FUNCTION "Gest Avvisi/Allarmi" : VOID
TITLE =GESTIONE ALLARMI / AVVISI
AUTHOR : MassimoZ
VERSION : 0.1

BEGIN
NETWORK
TITLE ======== Avvisi Generali =======



NETWORK
TITLE =Avviso: Manca Marcia Generale
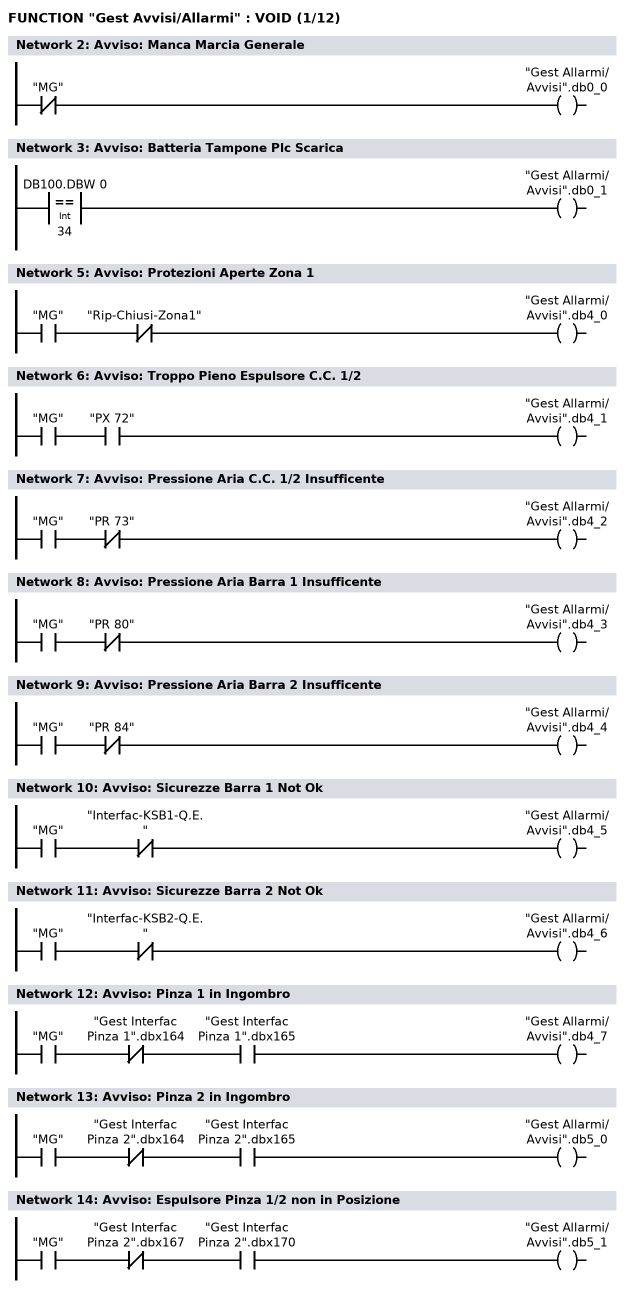
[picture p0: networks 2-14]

      UN    "MG";
      =     "Gest Allarmi/Avvisi".db0_0;
NETWORK
TITLE =Avviso: Batteria Tampone Plc Scarica

      L     DB100.DBW    0;
      L     34;
      ==I   ;
      =     "Gest Allarmi/Avvisi".db0_1;
NETWORK
TITLE ======== Avvisi Zona 1 =======



NETWORK
TITLE =Avviso: Protezioni Aperte Zona 1

      U     "MG";
      UN    "Rip-Chiusi-Zona1";
      =     "Gest Allarmi/Avvisi".db4_0;
NETWORK
TITLE =Avviso: Troppo Pieno Espulsore C.C. 1/2

      U     "MG";
      U     "PX 72";
      =     "Gest Allarmi/Avvisi".db4_1;
NETWORK
TITLE =Avviso: Pressione Aria C.C. 1/2 Insufficente

      U     "MG";
      UN    "PR 73";
      =     "Gest Allarmi/Avvisi".db4_2;
NETWORK
TITLE =Avviso: Pressione Aria Barra 1 Insufficente

      U     "MG";
      UN    "PR 80";
      =     "Gest Allarmi/Avvisi".db4_3;
NETWORK
TITLE =Avviso: Pressione Aria Barra 2 Insufficente

      U     "MG";
      UN    "PR 84";
      =     "Gest Allarmi/Avvisi".db4_4;
NETWORK
TITLE =Avviso: Sicurezze Barra 1 Not Ok

      U     "MG";
      UN    "Interfac-KSB1-Q.E.";
      =     "Gest Allarmi/Avvisi".db4_5;
NETWORK
TITLE =Avviso: Sicurezze Barra 2 Not Ok

      U     "MG";
      UN    "Interfac-KSB2-Q.E.";
      =     "Gest Allarmi/Avvisi".db4_6;
NETWORK
TITLE =Avviso: Pinza 1 in Ingombro

      U     "MG";
      UN    "Gest Interfac Pinza 1".dbx164;
      U     "Gest Interfac Pinza 1".dbx165;
      =     "Gest Allarmi/Avvisi".db4_7;
NETWORK
TITLE =Avviso: Pinza 2 in Ingombro

      U     "MG";
      UN    "Gest Interfac Pinza 2".dbx164;
      U     "Gest Interfac Pinza 2".dbx165;
      =     "Gest Allarmi/Avvisi".db5_0;
NETWORK
TITLE =Avviso: Espulsore Pinza 1/2 non in Posizione

      U     "MG";
      UN    "Gest Interfac Pinza 2".dbx167;
      U     "Gest Interfac Pinza 2".dbx170;
      =     "Gest Allarmi/Avvisi".db5_1;
NETWORK
TITLE =Avviso: Posa Coperchi in Ingombro
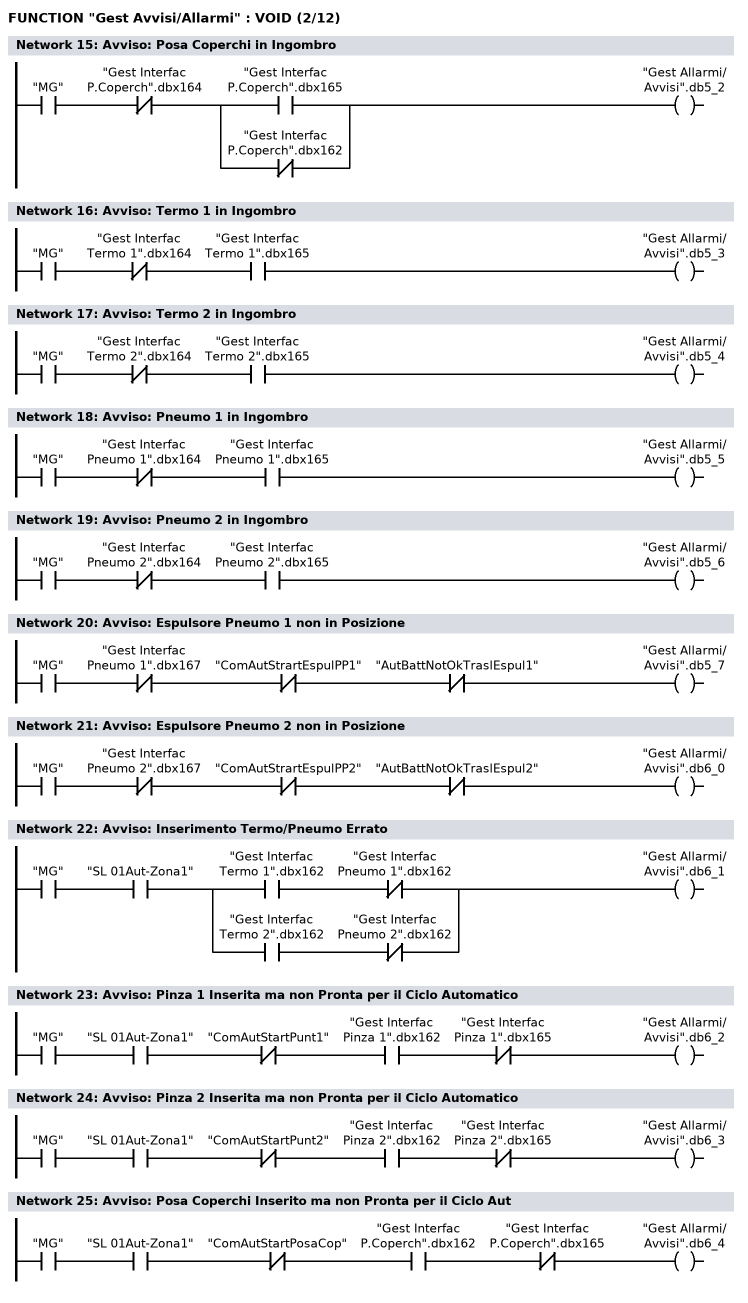
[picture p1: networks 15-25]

      U     "MG";
      UN    "Gest Interfac P.Coperch".dbx164;
      U(    ;
      O     "Gest Interfac P.Coperch".dbx165;
      ON    "Gest Interfac P.Coperch".dbx162;
      )     ;
      =     "Gest Allarmi/Avvisi".db5_2;
NETWORK
TITLE =Avviso: Termo 1 in Ingombro

      U     "MG";
      UN    "Gest Interfac Termo 1".dbx164;
      U     "Gest Interfac Termo 1".dbx165;
      =     "Gest Allarmi/Avvisi".db5_3;
NETWORK
TITLE =Avviso: Termo 2 in Ingombro

      U     "MG";
      UN    "Gest Interfac Termo 2".dbx164;
      U     "Gest Interfac Termo 2".dbx165;
      =     "Gest Allarmi/Avvisi".db5_4;
NETWORK
TITLE =Avviso: Pneumo 1 in Ingombro

      U     "MG";
      UN    "Gest Interfac Pneumo 1".dbx164;
      U     "Gest Interfac Pneumo 1".dbx165;
      =     "Gest Allarmi/Avvisi".db5_5;
NETWORK
TITLE =Avviso: Pneumo 2 in Ingombro

      U     "MG";
      UN    "Gest Interfac Pneumo 2".dbx164;
      U     "Gest Interfac Pneumo 2".dbx165;
      =     "Gest Allarmi/Avvisi".db5_6;
NETWORK
TITLE =Avviso: Espulsore Pneumo 1 non in Posizione

      U     "MG";
      UN    "Gest Interfac Pneumo 1".dbx167;
      UN    "ComAutStrartEspulPP1";
      UN    "AutBattNotOkTraslEspul1";
      =     "Gest Allarmi/Avvisi".db5_7;
NETWORK
TITLE =Avviso: Espulsore Pneumo 2 non in Posizione

      U     "MG";
      UN    "Gest Interfac Pneumo 2".dbx167;
      UN    "ComAutStrartEspulPP2";
      UN    "AutBattNotOkTraslEspul2";
      =     "Gest Allarmi/Avvisi".db6_0;
NETWORK
TITLE =Avviso: Inserimento Termo/Pneumo Errato

      U     "MG";
      U     "SL 01Aut-Zona1";
      U(    ;
      U     "Gest Interfac Termo 1".dbx162;
      UN    "Gest Interfac Pneumo 1".dbx162;
      O     ;
      U     "Gest Interfac Termo 2".dbx162;
      UN    "Gest Interfac Pneumo 2".dbx162;
      )     ;
      =     "Gest Allarmi/Avvisi".db6_1;
NETWORK
TITLE =Avviso: Pinza 1 Inserita ma non Pronta per il Ciclo Automatico

      U     "MG";
      U     "SL 01Aut-Zona1";
      UN    "ComAutStartPunt1";
      U     "Gest Interfac Pinza 1".dbx162;
      UN    "Gest Interfac Pinza 1".dbx165;
      =     "Gest Allarmi/Avvisi".db6_2;
NETWORK
TITLE =Avviso: Pinza 2 Inserita ma non Pronta per il Ciclo Automatico

      U     "MG";
      U     "SL 01Aut-Zona1";
      UN    "ComAutStartPunt2";
      U     "Gest Interfac Pinza 2".dbx162;
      UN    "Gest Interfac Pinza 2".dbx165;
      =     "Gest Allarmi/Avvisi".db6_3;
NETWORK
TITLE =Avviso: Posa Coperchi Inserito ma non Pronta per il Ciclo Aut

      U     "MG";
      U     "SL 01Aut-Zona1";
      UN    "ComAutStartPosaCop";
      U     "Gest Interfac P.Coperch".dbx162;
      UN    "Gest Interfac P.Coperch".dbx165;
      =     "Gest Allarmi/Avvisi".db6_4;
NETWORK
TITLE =Avviso: Termo 1 Inserita ma non Pronta per il Ciclo Automatico
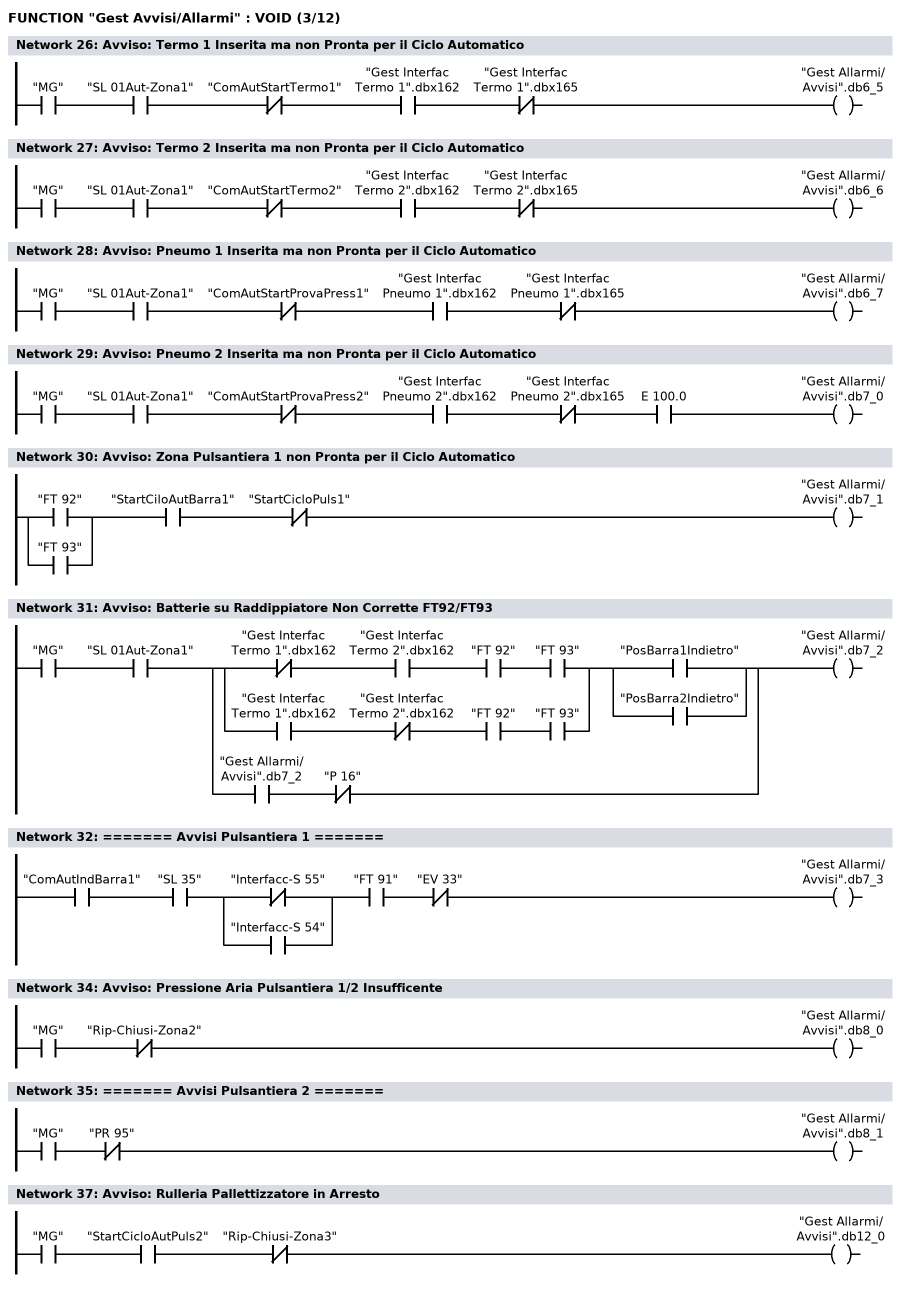
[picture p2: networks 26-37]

      U     "MG";
      U     "SL 01Aut-Zona1";
      UN    "ComAutStartTermo1";
      U     "Gest Interfac Termo 1".dbx162;
      UN    "Gest Interfac Termo 1".dbx165;
      =     "Gest Allarmi/Avvisi".db6_5;
NETWORK
TITLE =Avviso: Termo 2 Inserita ma non Pronta per il Ciclo Automatico

      U     "MG";
      U     "SL 01Aut-Zona1";
      UN    "ComAutStartTermo2";
      U     "Gest Interfac Termo 2".dbx162;
      UN    "Gest Interfac Termo 2".dbx165;
      =     "Gest Allarmi/Avvisi".db6_6;
NETWORK
TITLE =Avviso: Pneumo 1 Inserita ma non Pronta per il Ciclo Automatico

      U     "MG";
      U     "SL 01Aut-Zona1";
      UN    "ComAutStartProvaPress1";
      U     "Gest Interfac Pneumo 1".dbx162;
      UN    "Gest Interfac Pneumo 1".dbx165;
      =     "Gest Allarmi/Avvisi".db6_7;
NETWORK
TITLE =Avviso: Pneumo 2 Inserita ma non Pronta per il Ciclo Automatico

      U     "MG";
      U     "SL 01Aut-Zona1";
      UN    "ComAutStartProvaPress2";
      U     "Gest Interfac Pneumo 2".dbx162;
      UN    "Gest Interfac Pneumo 2".dbx165;
      U     E    100.0;
      =     "Gest Allarmi/Avvisi".db7_0;
NETWORK
TITLE =Avviso: Zona Pulsantiera 1 non Pronta per il Ciclo Automatico

      U(    ;
      O     "FT 92";
      O     "FT 93";
      )     ;
      U     "StartCiloAutBarra1";
      UN    "StartCicloPuls1";
      =     "Gest Allarmi/Avvisi".db7_1;
NETWORK
TITLE =Avviso: Batterie su Raddippiatore Non Corrette FT92/FT93

      U     "MG";
      U     "SL 01Aut-Zona1";
      U(    ;
      U(    ;
      UN    "Gest Interfac Termo 1".dbx162;
      U     "Gest Interfac Termo 2".dbx162;
      U     "FT 92";
      U     "FT 93";
      O     ;
      U     "Gest Interfac Termo 1".dbx162;
      UN    "Gest Interfac Termo 2".dbx162;
      U     "FT 92";
      U     "FT 93";
      )     ;
      U(    ;
      O     "PosBarra1Indietro";
      O     "PosBarra2Indietro";
      )     ;
      O     ;
      U     "Gest Allarmi/Avvisi".db7_2;
      UN    "P 16";
      )     ;
      =     "Gest Allarmi/Avvisi".db7_2;
NETWORK
TITLE ======== Avvisi Pulsantiera 1 =======



      U     "ComAutIndBarra1";
      U     "SL 35";
      U(    ;
      ON    "Interfacc-S 55";
      O     "Interfacc-S 54";
      )     ;
      U     "FT 91";
      UN    "EV 33";
      =     "Gest Allarmi/Avvisi".db7_3;
NETWORK
TITLE =Avviso: Protezioni Aperte Pulsantiera 1

NETWORK
TITLE =Avviso: Pressione Aria Pulsantiera 1/2 Insufficente

      U     "MG";
      UN    "Rip-Chiusi-Zona2";
      =     "Gest Allarmi/Avvisi".db8_0;
NETWORK
TITLE ======== Avvisi Pulsantiera 2 =======



      U     "MG";
      UN    "PR 95";
      =     "Gest Allarmi/Avvisi".db8_1;
NETWORK
TITLE =Avviso: Protezioni Aperte Pulsantiera 2

NETWORK
TITLE =Avviso: Rulleria Pallettizzatore in Arresto

      U     "MG";
      U     "StartCicloAutPuls2";
      UN    "Rip-Chiusi-Zona3";
      =     "Gest Allarmi/Avvisi".db12_0;
NETWORK
TITLE =Avviso: Troppo Pieno Rulleria Pallettizzatore
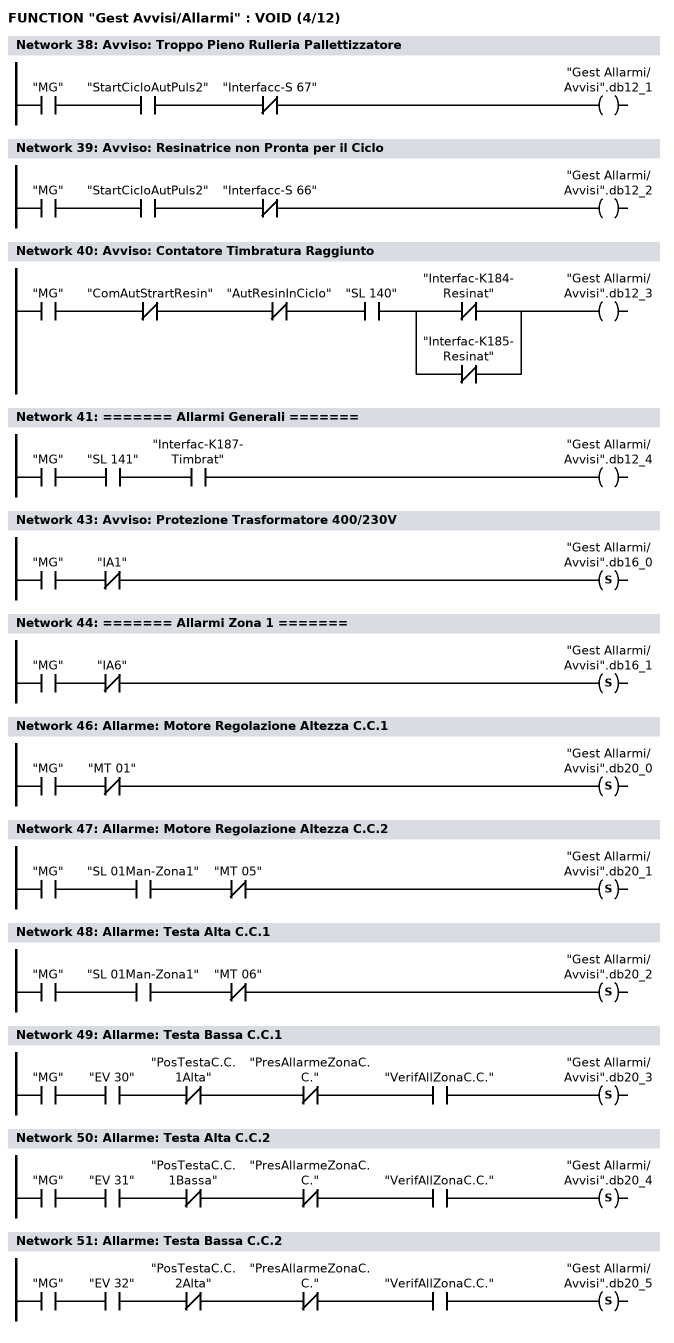
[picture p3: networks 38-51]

      U     "MG";
      U     "StartCicloAutPuls2";
      UN    "Interfacc-S 67";
      =     "Gest Allarmi/Avvisi".db12_1;
NETWORK
TITLE =Avviso: Resinatrice non Pronta per il Ciclo

      U     "MG";
      U     "StartCicloAutPuls2";
      UN    "Interfacc-S 66";
      =     "Gest Allarmi/Avvisi".db12_2;
NETWORK
TITLE =Avviso: Contatore Timbratura Raggiunto

      U     "MG";
      UN    "ComAutStrartResin";
      UN    "AutResinInCiclo";
      U     "SL 140";
      U(    ;
      ON    "Interfac-K184-Resinat";
      ON    "Interfac-K185-Resinat";
      )     ;
      =     "Gest Allarmi/Avvisi".db12_3;
NETWORK
TITLE ======== Allarmi Generali =======



      U     "MG";
      U     "SL 141";
      U     "Interfac-K187-Timbrat";
      =     "Gest Allarmi/Avvisi".db12_4;
NETWORK
TITLE =Avviso: Alimentazione Quadro Elettrico

NETWORK
TITLE =Avviso: Protezione Trasformatore 400/230V

      U     "MG";
      UN    "IA1";
      S     "Gest Allarmi/Avvisi".db16_0;
NETWORK
TITLE ======== Allarmi Zona 1 =======



      U     "MG";
      UN    "IA6";
      S     "Gest Allarmi/Avvisi".db16_1;
NETWORK
TITLE =Allarme: Motore Nastro 1

NETWORK
TITLE =Allarme: Motore Regolazione Altezza C.C.1

      U     "MG";
      UN    "MT 01";
      S     "Gest Allarmi/Avvisi".db20_0;
NETWORK
TITLE =Allarme: Motore Regolazione Altezza C.C.2

      U     "MG";
      U     "SL 01Man-Zona1";
      UN    "MT 05";
      S     "Gest Allarmi/Avvisi".db20_1;
NETWORK
TITLE =Allarme: Testa Alta C.C.1

      U     "MG";
      U     "SL 01Man-Zona1";
      UN    "MT 06";
      S     "Gest Allarmi/Avvisi".db20_2;
NETWORK
TITLE =Allarme: Testa Bassa C.C.1

      U     "MG";
      U     "EV 30";
      UN    "PosTestaC.C.1Alta";
      UN    "PresAllarmeZonaC.C.";
      U     "VerifAllZonaC.C.";
      S     "Gest Allarmi/Avvisi".db20_3;
NETWORK
TITLE =Allarme: Testa Alta C.C.2

      U     "MG";
      U     "EV 31";
      UN    "PosTestaC.C.1Bassa";
      UN    "PresAllarmeZonaC.C.";
      U     "VerifAllZonaC.C.";
      S     "Gest Allarmi/Avvisi".db20_4;
NETWORK
TITLE =Allarme: Testa Bassa C.C.2

      U     "MG";
      U     "EV 32";
      UN    "PosTestaC.C.2Alta";
      UN    "PresAllarmeZonaC.C.";
      U     "VerifAllZonaC.C.";
      S     "Gest Allarmi/Avvisi".db20_5;
NETWORK
TITLE =Allarme: Parzializzatore Inizio Linea Aperto
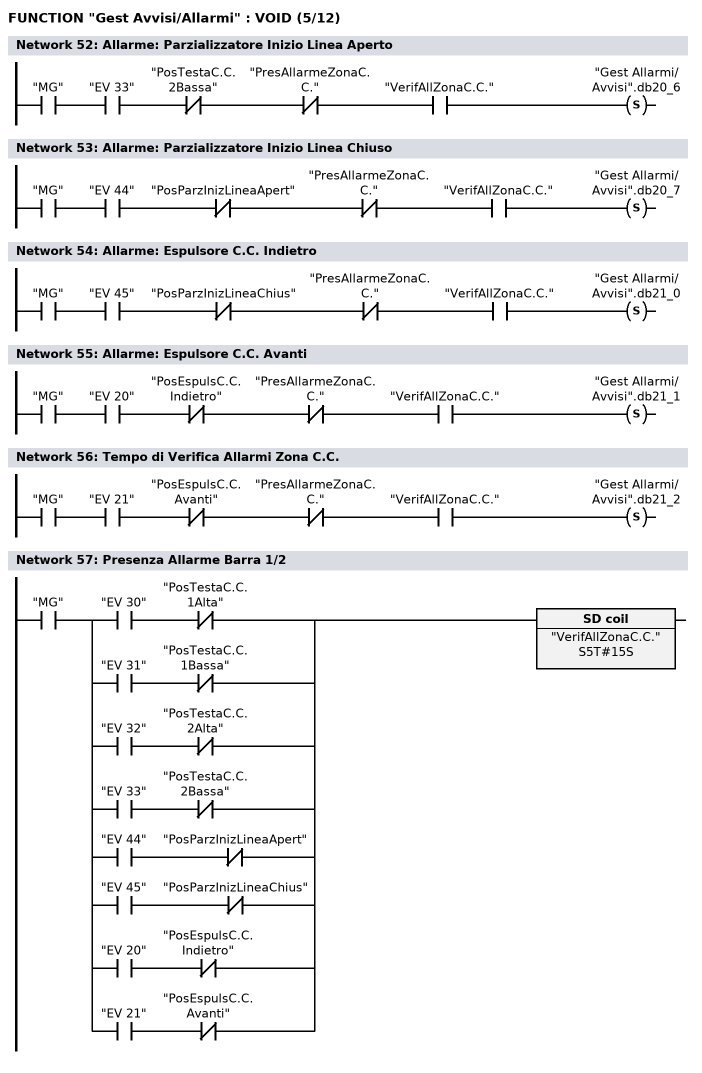
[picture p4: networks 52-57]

      U     "MG";
      U     "EV 33";
      UN    "PosTestaC.C.2Bassa";
      UN    "PresAllarmeZonaC.C.";
      U     "VerifAllZonaC.C.";
      S     "Gest Allarmi/Avvisi".db20_6;
NETWORK
TITLE =Allarme: Parzializzatore Inizio Linea Chiuso

      U     "MG";
      U     "EV 44";
      UN    "PosParzInizLineaApert";
      UN    "PresAllarmeZonaC.C.";
      U     "VerifAllZonaC.C.";
      S     "Gest Allarmi/Avvisi".db20_7;
NETWORK
TITLE =Allarme: Espulsore C.C. Indietro

      U     "MG";
      U     "EV 45";
      UN    "PosParzInizLineaChius";
      UN    "PresAllarmeZonaC.C.";
      U     "VerifAllZonaC.C.";
      S     "Gest Allarmi/Avvisi".db21_0;
NETWORK
TITLE =Allarme: Espulsore C.C. Avanti

      U     "MG";
      U     "EV 20";
      UN    "PosEspulsC.C.Indietro";
      UN    "PresAllarmeZonaC.C.";
      U     "VerifAllZonaC.C.";
      S     "Gest Allarmi/Avvisi".db21_1;
NETWORK
TITLE =Tempo di Verifica Allarmi Zona C.C.

      U     "MG";
      U     "EV 21";
      UN    "PosEspulsC.C.Avanti";
      UN    "PresAllarmeZonaC.C.";
      U     "VerifAllZonaC.C.";
      S     "Gest Allarmi/Avvisi".db21_2;
NETWORK
TITLE =Presenza Allarme Barra 1/2

      U     "MG";
      U(    ;
      U     "EV 30";
      UN    "PosTestaC.C.1Alta";
      O     ;
      U     "EV 31";
      UN    "PosTestaC.C.1Bassa";
      O     ;
      U     "EV 32";
      UN    "PosTestaC.C.2Alta";
      O     ;
      U     "EV 33";
      UN    "PosTestaC.C.2Bassa";
      O     ;
      U     "EV 44";
      UN    "PosParzInizLineaApert";
      O     ;
      U     "EV 45";
      UN    "PosParzInizLineaChius";
      O     ;
      U     "EV 20";
      UN    "PosEspulsC.C.Indietro";
      O     ;
      U     "EV 21";
      UN    "PosEspulsC.C.Avanti";
      )     ;
      L     S5T#15S;
      SE    "VerifAllZonaC.C.";
NETWORK
TITLE =Allarme: Barra 1 Indietro
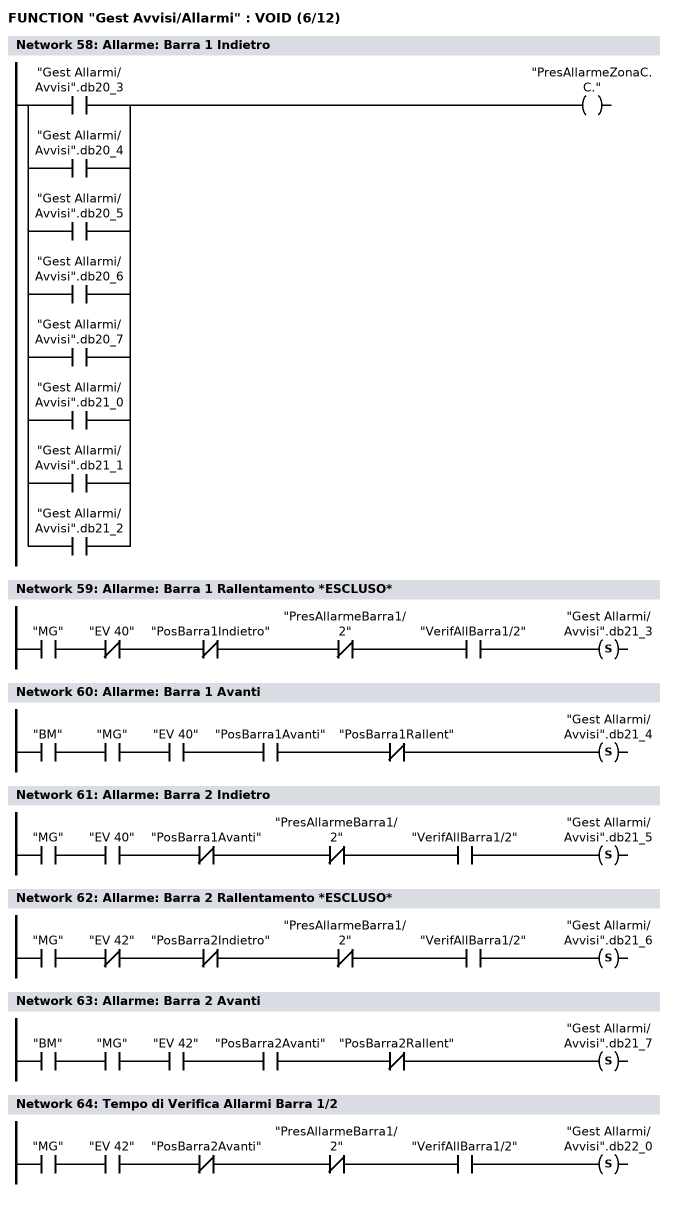
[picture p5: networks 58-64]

      O     "Gest Allarmi/Avvisi".db20_3;
      O     "Gest Allarmi/Avvisi".db20_4;
      O     "Gest Allarmi/Avvisi".db20_5;
      O     "Gest Allarmi/Avvisi".db20_6;
      O     "Gest Allarmi/Avvisi".db20_7;
      O     "Gest Allarmi/Avvisi".db21_0;
      O     "Gest Allarmi/Avvisi".db21_1;
      O     "Gest Allarmi/Avvisi".db21_2;
      =     "PresAllarmeZonaC.C.";
NETWORK
TITLE =Allarme: Barra 1 Rallentamento *ESCLUSO*

      U     "MG";
      UN    "EV 40";
      UN    "PosBarra1Indietro";
      UN    "PresAllarmeBarra1/2";
      U     "VerifAllBarra1/2";
      S     "Gest Allarmi/Avvisi".db21_3;
NETWORK
TITLE =Allarme: Barra 1 Avanti

      U     "BM";
      U     "MG";
      U     "EV 40";
      U     "PosBarra1Avanti";
      UN    "PosBarra1Rallent";
      S     "Gest Allarmi/Avvisi".db21_4;
NETWORK
TITLE =Allarme: Barra 2 Indietro

      U     "MG";
      U     "EV 40";
      UN    "PosBarra1Avanti";
      UN    "PresAllarmeBarra1/2";
      U     "VerifAllBarra1/2";
      S     "Gest Allarmi/Avvisi".db21_5;
NETWORK
TITLE =Allarme: Barra 2 Rallentamento *ESCLUSO*

      U     "MG";
      UN    "EV 42";
      UN    "PosBarra2Indietro";
      UN    "PresAllarmeBarra1/2";
      U     "VerifAllBarra1/2";
      S     "Gest Allarmi/Avvisi".db21_6;
NETWORK
TITLE =Allarme: Barra 2 Avanti

      U     "BM";
      U     "MG";
      U     "EV 42";
      U     "PosBarra2Avanti";
      UN    "PosBarra2Rallent";
      S     "Gest Allarmi/Avvisi".db21_7;
NETWORK
TITLE =Tempo di Verifica Allarmi Barra 1/2

      U     "MG";
      U     "EV 42";
      UN    "PosBarra2Avanti";
      UN    "PresAllarmeBarra1/2";
      U     "VerifAllBarra1/2";
      S     "Gest Allarmi/Avvisi".db22_0;
NETWORK
TITLE =Presenza Allarme Barra 1/2
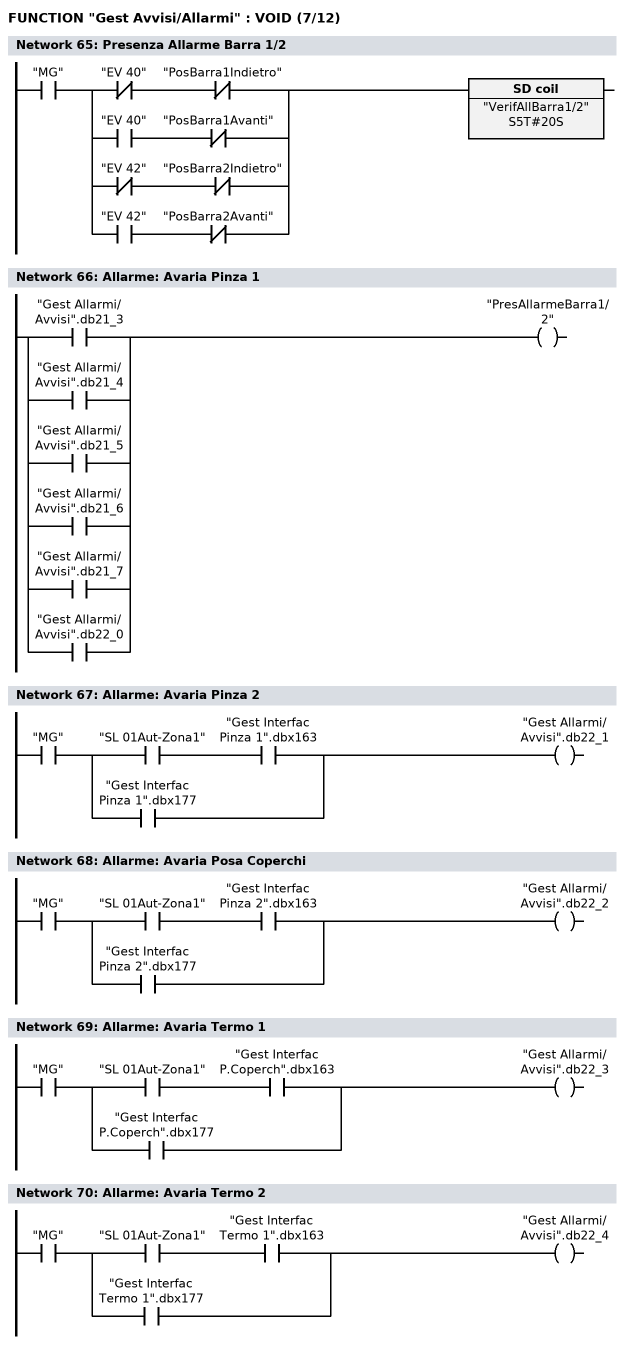
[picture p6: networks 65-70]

      U     "MG";
      U(    ;
      UN    "EV 40";
      UN    "PosBarra1Indietro";
      O     ;
      U     "EV 40";
      UN    "PosBarra1Avanti";
      O     ;
      UN    "EV 42";
      UN    "PosBarra2Indietro";
      O     ;
      U     "EV 42";
      UN    "PosBarra2Avanti";
      )     ;
      L     S5T#20S;
      SE    "VerifAllBarra1/2";
NETWORK
TITLE =Allarme: Avaria Pinza 1

      O     "Gest Allarmi/Avvisi".db21_3;
      O     "Gest Allarmi/Avvisi".db21_4;
      O     "Gest Allarmi/Avvisi".db21_5;
      O     "Gest Allarmi/Avvisi".db21_6;
      O     "Gest Allarmi/Avvisi".db21_7;
      O     "Gest Allarmi/Avvisi".db22_0;
      =     "PresAllarmeBarra1/2";
NETWORK
TITLE =Allarme: Avaria Pinza 2

      U     "MG";
      U(    ;
      U     "SL 01Aut-Zona1";
      U     "Gest Interfac Pinza 1".dbx163;
      O     "Gest Interfac Pinza 1".dbx177;
      )     ;
      =     "Gest Allarmi/Avvisi".db22_1;
NETWORK
TITLE =Allarme: Avaria Posa Coperchi

      U     "MG";
      U(    ;
      U     "SL 01Aut-Zona1";
      U     "Gest Interfac Pinza 2".dbx163;
      O     "Gest Interfac Pinza 2".dbx177;
      )     ;
      =     "Gest Allarmi/Avvisi".db22_2;
NETWORK
TITLE =Allarme: Avaria Termo 1

      U     "MG";
      U(    ;
      U     "SL 01Aut-Zona1";
      U     "Gest Interfac P.Coperch".dbx163;
      O     "Gest Interfac P.Coperch".dbx177;
      )     ;
      =     "Gest Allarmi/Avvisi".db22_3;
NETWORK
TITLE =Allarme: Avaria Termo 2

      U     "MG";
      U(    ;
      U     "SL 01Aut-Zona1";
      U     "Gest Interfac Termo 1".dbx163;
      O     "Gest Interfac Termo 1".dbx177;
      )     ;
      =     "Gest Allarmi/Avvisi".db22_4;
NETWORK
TITLE =Allarme: Avaria Pneumo 1
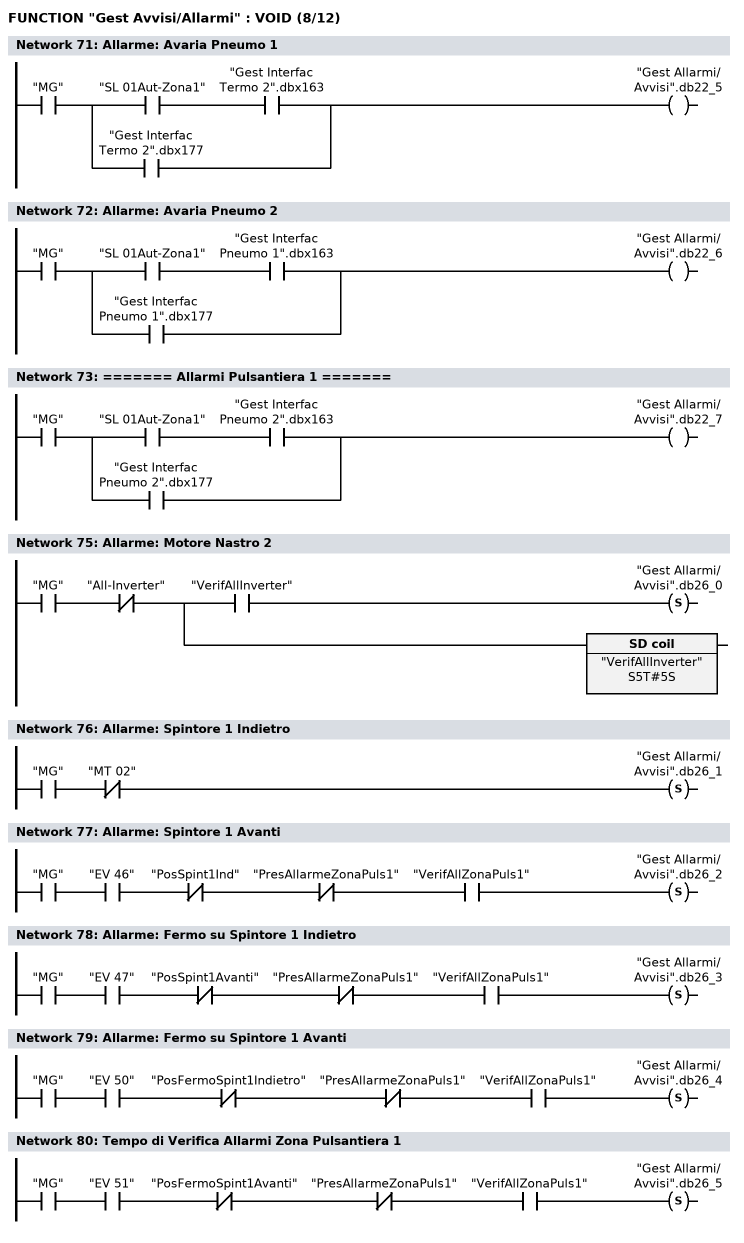
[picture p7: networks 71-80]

      U     "MG";
      U(    ;
      U     "SL 01Aut-Zona1";
      U     "Gest Interfac Termo 2".dbx163;
      O     "Gest Interfac Termo 2".dbx177;
      )     ;
      =     "Gest Allarmi/Avvisi".db22_5;
NETWORK
TITLE =Allarme: Avaria Pneumo 2

      U     "MG";
      U(    ;
      U     "SL 01Aut-Zona1";
      U     "Gest Interfac Pneumo 1".dbx163;
      O     "Gest Interfac Pneumo 1".dbx177;
      )     ;
      =     "Gest Allarmi/Avvisi".db22_6;
NETWORK
TITLE ======== Allarmi Pulsantiera 1 =======



      U     "MG";
      U(    ;
      U     "SL 01Aut-Zona1";
      U     "Gest Interfac Pneumo 2".dbx163;
      O     "Gest Interfac Pneumo 2".dbx177;
      )     ;
      =     "Gest Allarmi/Avvisi".db22_7;
NETWORK
TITLE =Allarme: Inverter

NETWORK
TITLE =Allarme: Motore Nastro 2

      U     "MG";
      UN    "All-Inverter";
      =     L      0.0;
      U     L      0.0;
      U     "VerifAllInverter";
      S     "Gest Allarmi/Avvisi".db26_0;
      U     L      0.0;
      BLD   102;
      L     S5T#5S;
      SE    "VerifAllInverter";
NETWORK
TITLE =Allarme: Spintore 1 Indietro

      U     "MG";
      UN    "MT 02";
      S     "Gest Allarmi/Avvisi".db26_1;
NETWORK
TITLE =Allarme: Spintore 1 Avanti

      U     "MG";
      U     "EV 46";
      UN    "PosSpint1Ind";
      UN    "PresAllarmeZonaPuls1";
      U     "VerifAllZonaPuls1";
      S     "Gest Allarmi/Avvisi".db26_2;
NETWORK
TITLE =Allarme: Fermo su Spintore 1 Indietro

      U     "MG";
      U     "EV 47";
      UN    "PosSpint1Avanti";
      UN    "PresAllarmeZonaPuls1";
      U     "VerifAllZonaPuls1";
      S     "Gest Allarmi/Avvisi".db26_3;
NETWORK
TITLE =Allarme: Fermo su Spintore 1 Avanti

      U     "MG";
      U     "EV 50";
      UN    "PosFermoSpint1Indietro";
      UN    "PresAllarmeZonaPuls1";
      U     "VerifAllZonaPuls1";
      S     "Gest Allarmi/Avvisi".db26_4;
NETWORK
TITLE =Tempo di Verifica Allarmi Zona Pulsantiera 1

      U     "MG";
      U     "EV 51";
      UN    "PosFermoSpint1Avanti";
      UN    "PresAllarmeZonaPuls1";
      U     "VerifAllZonaPuls1";
      S     "Gest Allarmi/Avvisi".db26_5;
NETWORK
TITLE =Presenza Allarme Zona Pulsantiera 1
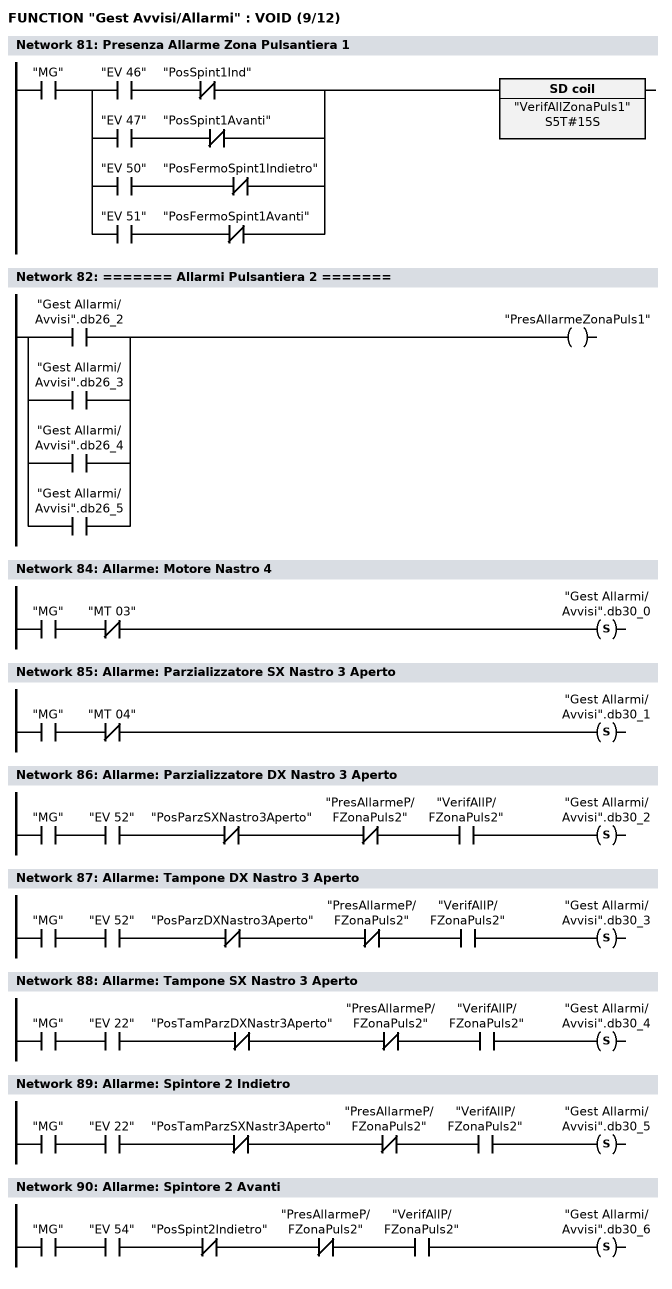
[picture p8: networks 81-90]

      U     "MG";
      U(    ;
      U     "EV 46";
      UN    "PosSpint1Ind";
      O     ;
      U     "EV 47";
      UN    "PosSpint1Avanti";
      O     ;
      U     "EV 50";
      UN    "PosFermoSpint1Indietro";
      O     ;
      U     "EV 51";
      UN    "PosFermoSpint1Avanti";
      )     ;
      L     S5T#15S;
      SE    "VerifAllZonaPuls1";
NETWORK
TITLE ======== Allarmi Pulsantiera 2 =======



      O     "Gest Allarmi/Avvisi".db26_2;
      O     "Gest Allarmi/Avvisi".db26_3;
      O     "Gest Allarmi/Avvisi".db26_4;
      O     "Gest Allarmi/Avvisi".db26_5;
      =     "PresAllarmeZonaPuls1";
NETWORK
TITLE =Allarme: Motore Nastro 3

NETWORK
TITLE =Allarme: Motore Nastro 4

      U     "MG";
      UN    "MT 03";
      S     "Gest Allarmi/Avvisi".db30_0;
NETWORK
TITLE =Allarme: Parzializzatore SX Nastro 3 Aperto

      U     "MG";
      UN    "MT 04";
      S     "Gest Allarmi/Avvisi".db30_1;
NETWORK
TITLE =Allarme: Parzializzatore DX Nastro 3 Aperto

      U     "MG";
      U     "EV 52";
      UN    "PosParzSXNastro3Aperto";
      UN    "PresAllarmeP/FZonaPuls2";
      U     "VerifAllP/FZonaPuls2";
      S     "Gest Allarmi/Avvisi".db30_2;
NETWORK
TITLE =Allarme: Tampone DX Nastro 3 Aperto

      U     "MG";
      U     "EV 52";
      UN    "PosParzDXNastro3Aperto";
      UN    "PresAllarmeP/FZonaPuls2";
      U     "VerifAllP/FZonaPuls2";
      S     "Gest Allarmi/Avvisi".db30_3;
NETWORK
TITLE =Allarme: Tampone SX Nastro 3 Aperto

      U     "MG";
      U     "EV 22";
      UN    "PosTamParzDXNastr3Aperto";
      UN    "PresAllarmeP/FZonaPuls2";
      U     "VerifAllP/FZonaPuls2";
      S     "Gest Allarmi/Avvisi".db30_4;
NETWORK
TITLE =Allarme: Spintore 2 Indietro

      U     "MG";
      U     "EV 22";
      UN    "PosTamParzSXNastr3Aperto";
      UN    "PresAllarmeP/FZonaPuls2";
      U     "VerifAllP/FZonaPuls2";
      S     "Gest Allarmi/Avvisi".db30_5;
NETWORK
TITLE =Allarme: Spintore 2 Avanti

      U     "MG";
      U     "EV 54";
      UN    "PosSpint2Indietro";
      UN    "PresAllarmeP/FZonaPuls2";
      U     "VerifAllP/FZonaPuls2";
      S     "Gest Allarmi/Avvisi".db30_6;
NETWORK
TITLE =Allarme: Fermo Anteriore Resinatrice Aperto
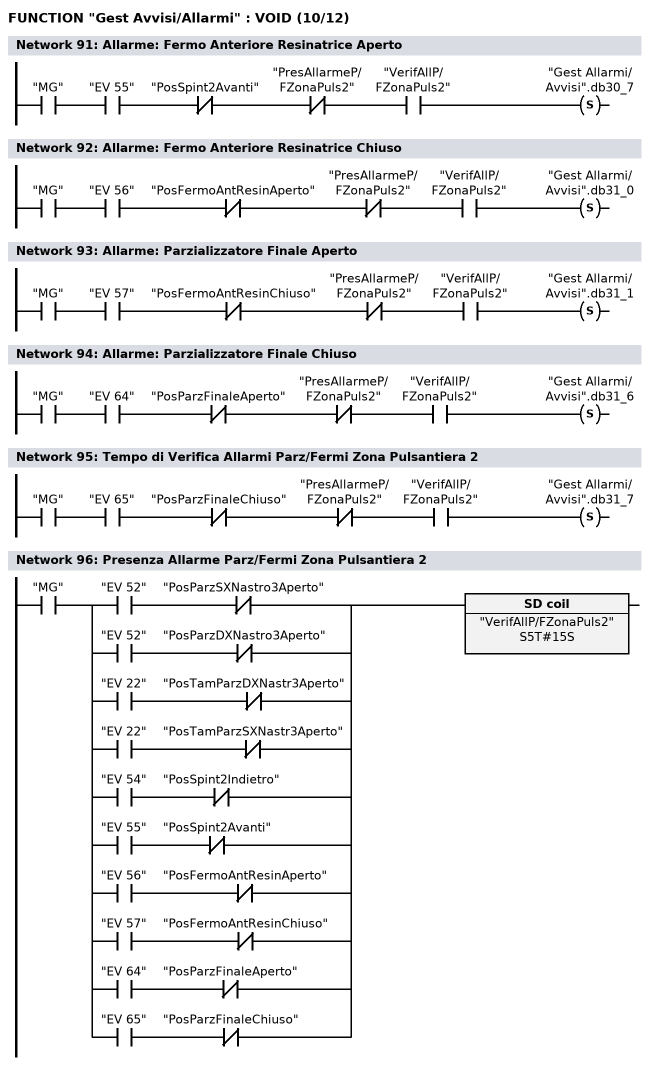
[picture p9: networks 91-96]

      U     "MG";
      U     "EV 55";
      UN    "PosSpint2Avanti";
      UN    "PresAllarmeP/FZonaPuls2";
      U     "VerifAllP/FZonaPuls2";
      S     "Gest Allarmi/Avvisi".db30_7;
NETWORK
TITLE =Allarme: Fermo Anteriore Resinatrice Chiuso

      U     "MG";
      U     "EV 56";
      UN    "PosFermoAntResinAperto";
      UN    "PresAllarmeP/FZonaPuls2";
      U     "VerifAllP/FZonaPuls2";
      S     "Gest Allarmi/Avvisi".db31_0;
NETWORK
TITLE =Allarme: Parzializzatore Finale Aperto

      U     "MG";
      U     "EV 57";
      UN    "PosFermoAntResinChiuso";
      UN    "PresAllarmeP/FZonaPuls2";
      U     "VerifAllP/FZonaPuls2";
      S     "Gest Allarmi/Avvisi".db31_1;
NETWORK
TITLE =Allarme: Parzializzatore Finale Chiuso

      U     "MG";
      U     "EV 64";
      UN    "PosParzFinaleAperto";
      UN    "PresAllarmeP/FZonaPuls2";
      U     "VerifAllP/FZonaPuls2";
      S     "Gest Allarmi/Avvisi".db31_6;
NETWORK
TITLE =Tempo di Verifica Allarmi Parz/Fermi Zona Pulsantiera 2

      U     "MG";
      U     "EV 65";
      UN    "PosParzFinaleChiuso";
      UN    "PresAllarmeP/FZonaPuls2";
      U     "VerifAllP/FZonaPuls2";
      S     "Gest Allarmi/Avvisi".db31_7;
NETWORK
TITLE =Presenza Allarme Parz/Fermi Zona Pulsantiera 2

      U     "MG";
      U(    ;
      U     "EV 52";
      UN    "PosParzSXNastro3Aperto";
      O     ;
      U     "EV 52";
      UN    "PosParzDXNastro3Aperto";
      O     ;
      U     "EV 22";
      UN    "PosTamParzDXNastr3Aperto";
      O     ;
      U     "EV 22";
      UN    "PosTamParzSXNastr3Aperto";
      O     ;
      U     "EV 54";
      UN    "PosSpint2Indietro";
      O     ;
      U     "EV 55";
      UN    "PosSpint2Avanti";
      O     ;
      U     "EV 56";
      UN    "PosFermoAntResinAperto";
      O     ;
      U     "EV 57";
      UN    "PosFermoAntResinChiuso";
      O     ;
      U     "EV 64";
      UN    "PosParzFinaleAperto";
      O     ;
      U     "EV 65";
      UN    "PosParzFinaleChiuso";
      )     ;
      L     S5T#15S;
      SE    "VerifAllP/FZonaPuls2";
NETWORK
TITLE =Allarme: Fermo Resinatrice Aperto
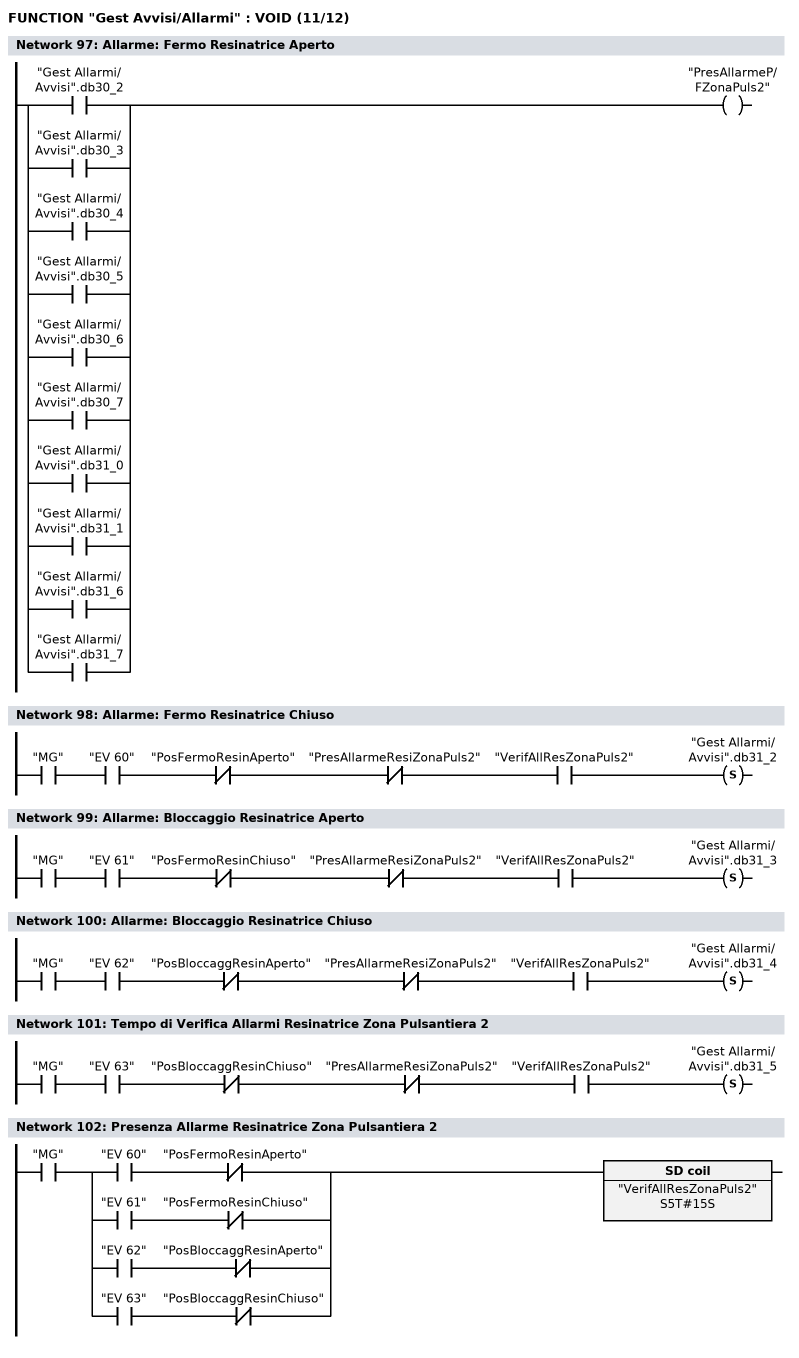
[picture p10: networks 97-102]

      O     "Gest Allarmi/Avvisi".db30_2;
      O     "Gest Allarmi/Avvisi".db30_3;
      O     "Gest Allarmi/Avvisi".db30_4;
      O     "Gest Allarmi/Avvisi".db30_5;
      O     "Gest Allarmi/Avvisi".db30_6;
      O     "Gest Allarmi/Avvisi".db30_7;
      O     "Gest Allarmi/Avvisi".db31_0;
      O     "Gest Allarmi/Avvisi".db31_1;
      O     "Gest Allarmi/Avvisi".db31_6;
      O     "Gest Allarmi/Avvisi".db31_7;
      =     "PresAllarmeP/FZonaPuls2";
NETWORK
TITLE =Allarme: Fermo Resinatrice Chiuso

      U     "MG";
      U     "EV 60";
      UN    "PosFermoResinAperto";
      UN    "PresAllarmeResiZonaPuls2";
      U     "VerifAllResZonaPuls2";
      S     "Gest Allarmi/Avvisi".db31_2;
NETWORK
TITLE =Allarme: Bloccaggio Resinatrice Aperto

      U     "MG";
      U     "EV 61";
      UN    "PosFermoResinChiuso";
      UN    "PresAllarmeResiZonaPuls2";
      U     "VerifAllResZonaPuls2";
      S     "Gest Allarmi/Avvisi".db31_3;
NETWORK
TITLE =Allarme: Bloccaggio Resinatrice Chiuso

      U     "MG";
      U     "EV 62";
      UN    "PosBloccaggResinAperto";
      UN    "PresAllarmeResiZonaPuls2";
      U     "VerifAllResZonaPuls2";
      S     "Gest Allarmi/Avvisi".db31_4;
NETWORK
TITLE =Tempo di Verifica Allarmi Resinatrice Zona Pulsantiera 2

      U     "MG";
      U     "EV 63";
      UN    "PosBloccaggResinChiuso";
      UN    "PresAllarmeResiZonaPuls2";
      U     "VerifAllResZonaPuls2";
      S     "Gest Allarmi/Avvisi".db31_5;
NETWORK
TITLE =Presenza Allarme Resinatrice Zona Pulsantiera 2

      U     "MG";
      U(    ;
      U     "EV 60";
      UN    "PosFermoResinAperto";
      O     ;
      U     "EV 61";
      UN    "PosFermoResinChiuso";
      O     ;
      U     "EV 62";
      UN    "PosBloccaggResinAperto";
      O     ;
      U     "EV 63";
      UN    "PosBloccaggResinChiuso";
      )     ;
      L     S5T#15S;
      SE    "VerifAllResZonaPuls2";
NETWORK
TITLE =Allarme: Avaria Resinatrice
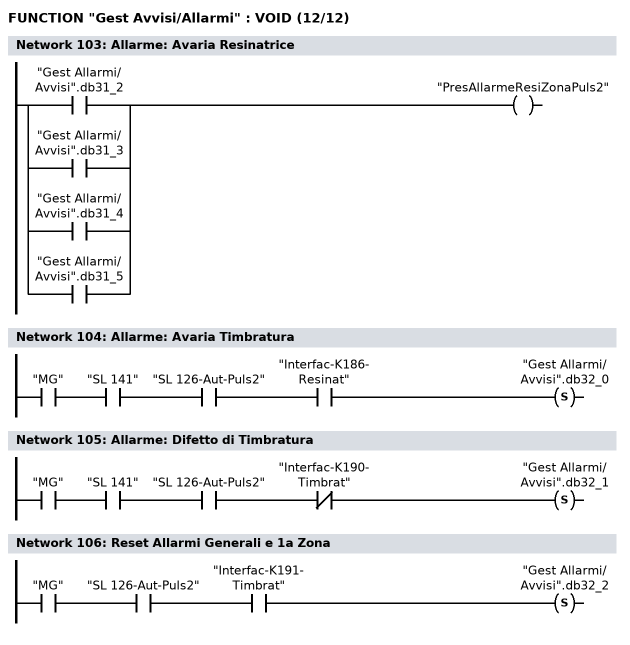
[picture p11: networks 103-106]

      O     "Gest Allarmi/Avvisi".db31_2;
      O     "Gest Allarmi/Avvisi".db31_3;
      O     "Gest Allarmi/Avvisi".db31_4;
      O     "Gest Allarmi/Avvisi".db31_5;
      =     "PresAllarmeResiZonaPuls2";
NETWORK
TITLE =Allarme: Avaria Timbratura

      U     "MG";
      U     "SL 141";
      U     "SL 126-Aut-Puls2";
      U     "Interfac-K186-Resinat";
      S     "Gest Allarmi/Avvisi".db32_0;
NETWORK
TITLE =Allarme: Difetto di Timbratura

      U     "MG";
      U     "SL 141";
      U     "SL 126-Aut-Puls2";
      UN    "Interfac-K190-Timbrat";
      S     "Gest Allarmi/Avvisi".db32_1;
NETWORK
TITLE =Reset Allarmi Generali e 1a Zona

      U     "MG";
      U     "SL 126-Aut-Puls2";
      U     "Interfac-K191-Timbrat";
      S     "Gest Allarmi/Avvisi".db32_2;
NETWORK
TITLE =Reset Allarmi Pulsantiera 1

      U     "P 16";
      FP    DB100.DBX   12.0;
      SPBNB M001;
      L     0;
      T     DB90.DBW   16;
      T     "Gest Allarmi/Avvisi".dbw18;
      T     DB90.DBW   20;

//ACQUISIZIONE ALLARMI DA PLC
//----------
      T     DB90.DBW   22;
      T     "Gest Allarmi/Avvisi".dbw24;
M001: NOP   0;
//----------
      L     DB90.DBW   16;
      INVI  ;
      T     DB90.DBW   36;
//----------
      L     "Gest Allarmi/Avvisi".dbw18;
      INVI  ;
      T     DB90.DBW   38;
      L     DB90.DBW   20;
      INVI  ;
      T     DB90.DBW   40;
      L     DB90.DBW   22;
      INVI  ;
      T     DB90.DBW   42;
      L     "Gest Allarmi/Avvisi".dbw24;
      INVI  ;
      T     "Gest Allarmi/Avvisi".dbw44;
NETWORK
TITLE =Reset Allarmi Pulsantiera 2

      U     "P 104";
      FP    DB100.DBX   12.1;
      SPBNB M002;
      L     0;
      T     DB90.DBW   26;
      T     "Gest Allarmi/Avvisi".dbw28;
M002: NOP   0;
      L     DB90.DBW   26;

//ACQUISIZIONE ALLARMI DA PLC
//----------
      INVI  ;
      T     DB90.DBW   46;
      L     "Gest Allarmi/Avvisi".dbw28;
//----------
      INVI  ;
      T     DB90.DBW   48;
NETWORK
TITLE =

      U     "P 134";
      FP    DB100.DBX   12.2;
      SPBNB M003;
      L     0;
      T     DB90.DBW   30;
      T     DB90.DBW   32;
      T     "Gest Allarmi/Avvisi".dbw34;
M003: NOP   0;
      L     DB90.DBW   30;
      INVI  ;
      T     DB90.DBW   50;
      L     DB90.DBW   32;
      INVI  ;
      T     DB90.DBW   52;
      L     "Gest Allarmi/Avvisi".dbw34;
      INVI  ;
      T     "Gest Allarmi/Avvisi".dbw54;
END_FUNCTION

